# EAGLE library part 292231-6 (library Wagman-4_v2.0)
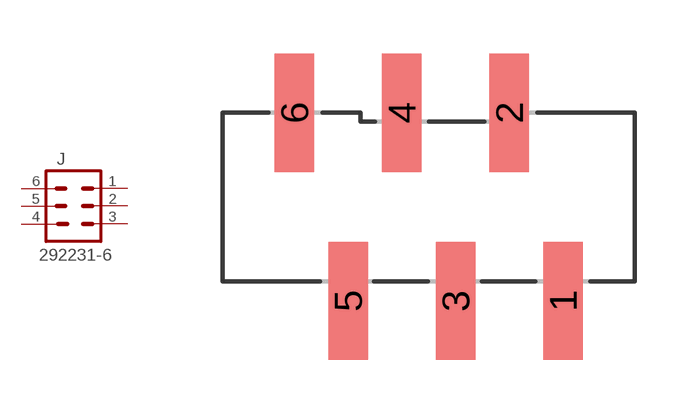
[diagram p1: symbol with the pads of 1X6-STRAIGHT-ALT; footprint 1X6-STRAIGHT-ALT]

Designator prefix J

## 292231-6  [1X6-STRAIGHT-ALT]
1  1  pas
2  2  pas
3  3  pas
4  4  pas
5  5  pas
6  6  pas

## Footprint 1X6-STRAIGHT-ALT (pad centres in mm)
smd 1.1 x 3.3: 1 3.75,-2.9; 2 2.25,2.35; 3 0.75,-2.9; 4 -0.75,2.35; 5 -2.25,-2.9; 6 -3.75,2.35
